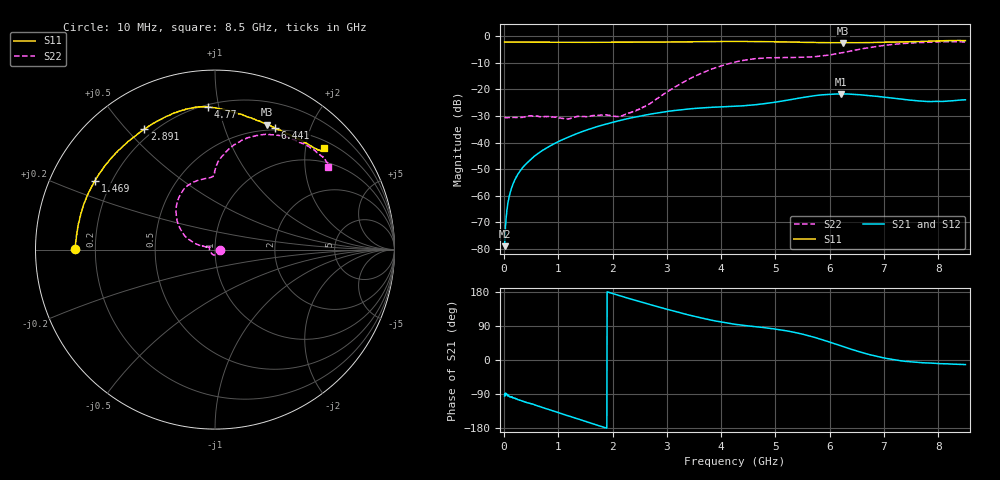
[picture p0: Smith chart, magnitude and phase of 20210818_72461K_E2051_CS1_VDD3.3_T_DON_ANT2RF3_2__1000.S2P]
!Agilent Technologies,E5071C,MY46417908,A.11.23
!Date: Wed Aug 18 14:29:17 2021
!Data & Calibration Information:
!Freq	S11:SOLT2(ON)	S21:SOLT2(ON)	S12:SOLT2(ON)	S22:SOLT2(ON)
!PortZ  Port1:50+j0  Port2:50+j0
!Above PortZ is port z conversion or system Z0 setting when saving the data.
!When reading, reference impedance value at option line is always used.
# Hz S dB R 50
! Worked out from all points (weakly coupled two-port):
!   1601 points, 10 MHz to 8.5 GHz, reference 50 ohm
!   highest |S21| = -21.68 dB at 6.208 GHz (marker M1); lowest = -78.9 dB at 10 MHz (marker M2)
!   lowest |S11| = -2.5 dB at 6.25 GHz (marker M3), VSWR 7.09, Z = 21.8 + j70.1 ohm
!   |S11| at or under -10 dB: nowhere
!   |S22| runs from -31.1 to -2.0 dB; largest |S21 - S12| = 0.00033
!   S11 on the Smith chart (normalised r, x): 10 MHz: 0.12, +0.00; 1.469 GHz: 0.14, +0.26; 2.891 GHz: 0.17, +0.56; 4.77 GHz: 0.21, +0.93; 6.441 GHz: 0.48, +1.50; 8.5 GHz: 0.65, +2.38
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1e7  -2.14 179.7  -78.94 -94.9  -81.18 -92.1  -30.39 -2.1
6.836875e7  -2.18 178.5  -62.96 -91.1  -63.29 -92.8  -30.60 -7.9
1.108188e8  -2.18 177.6  -58.90 -96.8  -58.97 -95.8  -30.54 -11.6
1.957188e8  -2.20 175.9  -54.08 -100.6  -54.11 -101.6  -30.48 -20.9
3.124562e8  -2.22 173.4  -50.23 -107.3  -50.17 -107.1  -30.54 -37.5
7.3165e8  -2.23 164.8  -42.65 -126.5  -42.64 -126.4  -30.23 -90.7
1.150844e9  -2.24 156.5  -38.19 -146.0  -38.23 -145.9  -31.07 -144.5
1.426769e9  -2.26 151.0  -35.94 -158.6  -35.97 -158.5  -30.15 -175.3
1.469219e9  -2.26 150.1  -35.63 -160.5  -35.65 -160.5  -30.21 -179.3
2.153725e9  -2.26 136.0  -31.57 168.7  -31.58 168.7  -30.04 154.9
2.843538e9  -2.19 121.4  -28.78 140.1  -28.79 140.1  -23.10 163.8
2.891294e9  -2.19 120.4  -28.63 138.2  -28.64 138.2  -22.44 164.0
3.512125e9  -2.04 109.3  -27.13 115.0  -27.13 115.0  -15.04 156.6
4.255e9  -1.94 98.8  -26.29 94.3  -26.31 94.3  -9.71 130.9
4.769706e9  -1.99 92.7  -25.41 85.8  -25.41 85.8  -8.19 111.8
5.671769e9  -2.30 78.9  -22.50 61.7  -22.50 61.8  -7.74 91.2
6.2077e9  -2.43 68.6  -21.68 37.4  -21.70 37.3  -6.23 88.2
6.25015e9  -2.47 67.6  -21.71 35.3  -21.73 35.2  -6.10 87.5
6.441175e9  -2.44 63.7  -21.85 26.4  -21.86 26.2  -5.31 84.0
7.088538e9  -2.20 51.4  -23.10 3.1  -23.12 2.9  -3.21 67.9
7.937538e9  -1.76 42.4  -24.49 -8.7  -24.48 -8.7  -2.12 44.9
8.5e9  -1.62 43.1  -23.90 -12.1  -23.89 -12.3  -2.14 36.1
